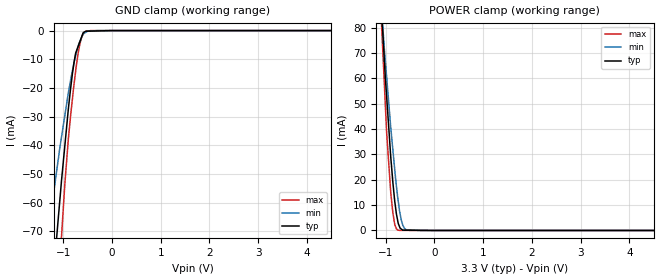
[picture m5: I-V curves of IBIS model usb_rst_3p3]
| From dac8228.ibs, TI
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|   usb_rst_3p3 Model
[Model]   usb_rst_3p3
Model_type   Input
Vinl = 0.6
Vinh = 2.3
|   typ   min   max
|   (nom PVT)   (Fast PVT)   (slow PVT)
|C_comp from frequency method(F=50MHz)
|Average
|C_comp   9.267e-12   7.756e-12   1.070e-11
|C_comp from L-C Tank method(L=1nH)
|Resonant Frequency(Hz)   1.72e9   1.86e9   1.61e9
C_comp   8.571e-12   7.329e-12   9.782e-12
| Where nom  PVT is Nominal Process,  3.3V,  33C
|   Fast PVT is Strong Process,   3.6V,  -40C
|   Slow PVT is Weak Process,   3V,  113C
[Voltage Range]   3.3   3   3.6
|Ambient Temperature   25   105   -40
|Junction Temperature
[Temperature Range]   33   113   -40
[Power Clamp Reference]   3.3   3   3.6
[GND Clamp Reference]   0   0   0
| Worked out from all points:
|   GND clamp passes 1 mA (typ) near -0.60 V on its own axis
|   POWER clamp passes 1 mA (typ) near -0.71 V on its own axis
[GND Clamp]
|   Voltage   I(typ)   I(min)   I(max)
-3.3V     -572.7mA   -387.4mA   -802.2mA
-1.361V   -118.9mA   -77.73mA   -170.9mA
-1.272V   -100mA     -65.91mA   -143mA
-1.184V   -81.73mA   -55mA      -115.6mA
-1.071V   -59.2mA    -40.91mA   -81.77mA
-1.036V   -52.29mA   -37.09mA   -71.86mA
-896.4mV  -27.44mA   -21.78mA   -37.88mA
-811.8mV  -14.96mA   -13.98mA   -23.71mA
-738mV    -7.483mA   -8.126mA   -12.99mA
-655.2mV  -3.679mA   -3.589mA   -4.387mA
-537.9mV  -215.9uA   -600.8uA   -323.7uA
6.6V      0A         0A         0A
[POWER Clamp]
|   Voltage   I(typ)   I(min)   I(max)
-3.3V     869.3mA    734.6mA    1.044A
-1.084V   85.81mA    86.41mA    79.97mA
-1.032V   68.16mA    72.24mA    58.91mA
-982.8mV  52.97mA    60.65mA    38.83mA
-896.4mV  28.7mA     40.32mA    14.56mA
-853.2mV  18.73mA    31.56mA    6.771mA
-817.2mV  11.76mA    24.27mA    2.531mA
-756mV    3.952mA    13.19mA    210.4uA
-687mV    641.4uA    4.545mA    38.04uA
-651mV    146.4uA    2.075mA    32.51uA
-573mV    128.8uA    253uA      20.54uA
6.6V      0A         0A         0A
